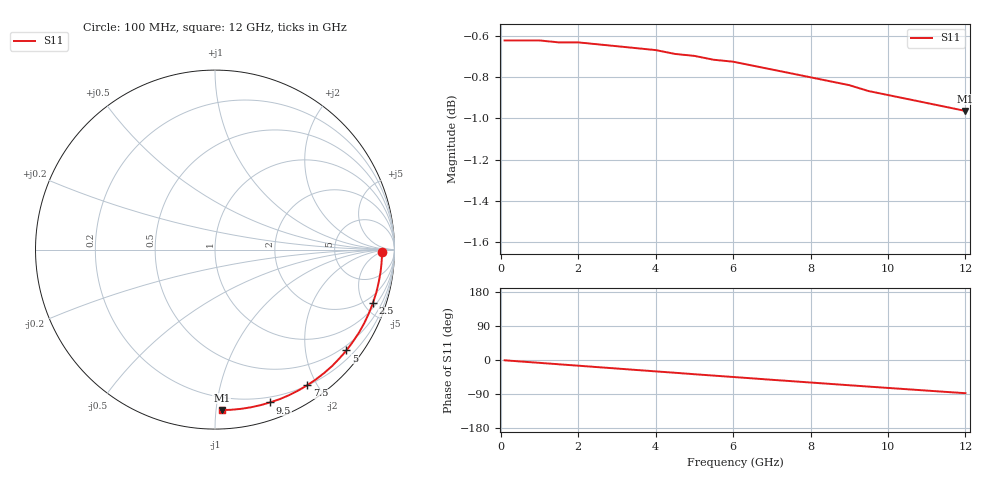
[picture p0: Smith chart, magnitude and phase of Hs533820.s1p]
!HSCH-5318 and HSCH-5338 Schottky diodes
!S-parameters at 20 microamps external bias.  Last updated 6/7/94
# ghz s ma r 50
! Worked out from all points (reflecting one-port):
!   25 points, 100 MHz to 12 GHz, reference 50 ohm
!   lowest |S11| = -1.0 dB at 12 GHz (marker M1), VSWR 18.05, Z = 5.76 - j51.8 ohm
!   phase of S11 starts at -1 deg and turns -87 deg over the sweep
!   S11 on the Smith chart (normalised r, x): 100 MHz: 27, -5; 2.5 GHz: 1.31, -5.75; 5 GHz: 0.38, -2.90; 7.5 GHz: 0.20, -1.87; 9.5 GHz: 0.15, -1.41; 12 GHz: 0.12, -1.04
0.1  0.931 -0.8
0.5  0.931 -3.8
1  0.931 -7.5
1.5  0.93 -11.3
2  0.93 -15.0
2.5  0.929 -18.8
3  0.928 -22.5
3.5  0.927 -26.3
4  0.926 -30.0
4.5  0.924 -33.7
5  0.923 -37.5
5.5  0.921 -41.2
6  0.92 -44.8
6.5  0.918 -48.5
7  0.916 -52.2
7.5  0.914 -55.8
8  0.912 -59.4
8.5  0.91 -63.0
9  0.908 -66.6
9.5  0.905 -70.2
10  0.903 -73.7
10.5  0.901 -77.2
11  0.899 -80.7
11.5  0.897 -84.2
12  0.895 -87.6
